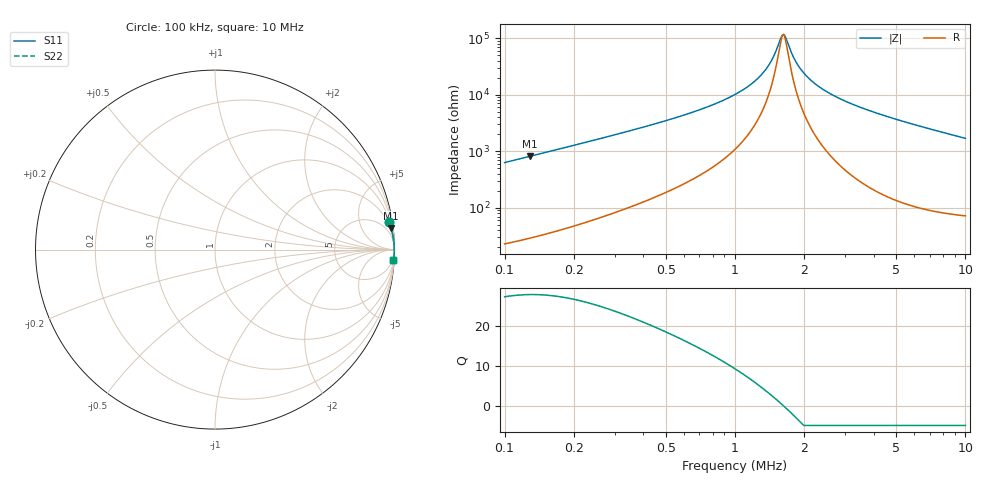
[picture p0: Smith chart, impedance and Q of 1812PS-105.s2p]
# MHz S MA R 50
!Freq  MagS11  AngS11  MagS21  AngS21  MagS12  AngS12  MagS22  AngS22
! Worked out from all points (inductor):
!   801 points, 100 kHz to 10 MHz, reference 50 ohm
!   read as one part in series: L = 999 uH near 102.3 kHz
!   highest Q = 28 at 128.8 kHz (marker M1), where L = 1.01 mH
!   self-resonance near 1.613 MHz
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0.1  0.9822 9.0  0.1557 -79.0  0.1557 -79.0  0.9822 9.0
0.128825  0.9883 7.0  0.1213 -81.0  0.1213 -81.0  0.9883 7.0
0.2385064  0.9954 3.7  0.065 -84.0  0.065 -84.0  0.9954 3.7
0.4004055  0.9975 2.1  0.03726 -85.1  0.03726 -85.1  0.9975 2.1
0.5821032  0.9983 1.4  0.02381 -85.2  0.02381 -85.2  0.9983 1.4
1.065369  0.9989 0.5  0.008531 -82.6  0.008531 -82.6  0.9989 0.5
1.28825  0.999 0.3  0.004635 -78.0  0.004635 -78.0  0.999 0.3
1.437143  0.9991 0.1  0.002524 -69.0  0.002524 -69.0  0.9991 0.1
1.575796  0.9991 0.0  0.001025 -32.1  0.001025 -32.1  0.9991 0.0
1.603245  0.9991 0.0  0.0008866 -13.4  0.0008866 -13.4  0.9991 0.0
1.650061  0.9991 -0.0  0.0009258 22.8  0.0009258 22.8  0.9991 -0.0
1.757924  0.9992 -0.1  0.001808 62.4  0.001808 62.4  0.9992 -0.1
1.851399  0.9992 -0.2  0.002752 72.5  0.002752 72.5  0.9992 -0.2
1.961101  0.9992 -0.2  0.003857 77.7  0.003857 77.7  0.9992 -0.2
2.101358  0.9992 -0.3  0.005223 80.9  0.005223 80.9  0.9992 -0.3
2.277718  0.9992 -0.4  0.006861 83.0  0.006861 83.0  0.9992 -0.4
2.754229  0.9992 -0.6  0.01094 85.3  0.01094 85.3  0.9992 -0.6
3.408003  0.9991 -0.9  0.01599 86.2  0.01599 86.2  0.9991 -0.9
5.069907  0.9986 -1.6  0.02757 86.3  0.02757 86.3  0.9986 -1.6
6.722023  0.9979 -2.2  0.03831 85.8  0.03831 85.8  0.9979 -2.2
8.365656  0.9969 -2.8  0.04866 85.0  0.04866 85.0  0.9969 -2.8
10  0.9958 -3.4  0.05876 84.2  0.05876 84.2  0.9958 -3.4
